PROGRAM BATH
VAR	
	fbLight1: FB_Light;
	
	R_TRIG_BlindUp: R_TRIG;	
	R_TRIG_BlindDown: R_TRIG;
	bSwitchBlindUp: BOOL;
	bSwitchBlindDown: BOOL;
	fbVenetianBlind: FB_VenetianBlind;	
END_VAR
VAR_OUTPUT
	rTemperature: LREAL;
END_VAR

// Light 1
fbLight1(bOn:= , bOff:= , bToggle:= GVL.I_bTerm2_Var14, bLight=> GVL.Q_bTerm4_Var4);
		
// Blind 1
R_TRIG_BlindUp(CLK:=GVL.I_bTerm2_Var15);
bSwitchBlindUp:=R_TRIG_BlindUp.Q;
R_TRIG_BlindDown(CLK:=GVL.I_bTerm2_Var16);
bSwitchBlindDown:= R_TRIG_BlindDown.Q;

fbVenetianBlind(
	bUp:= bSwitchBlindUp, 
	bDown:= bSwitchBlindDown, 
	bStop:= (bSwitchBlindUp OR bSwitchBlindDown) AND (fbVenetianBlind.bBlindUp OR fbVenetianBlind.bBlindDown), 
	bSwitchOverUp:= , 
	bSwitchOverDown:= , 
	tSwitchOverTime:= , 
	bStepUp:= , 
	bStepDown:= , 
	tStepTime:= , 
	bShadowPosition:= , 
	tShadowTurnAroundTime:= , 
	tShadowTurnOffTime:= , 
	bSafetyPosition:= , 
	tTurnOffTime:= , 
	tSwitchOverDeadTime:= , 
	bBlindUp=> GVL.Q_bTerm12_Var1, 
	bBlindDown=> GVL.Q_bTerm12_Var2);
	
	
// Temperature
rTemperature := INT_TO_LREAL(GVL.I_nTerm5_Var1) / 10;

END_PROGRAM
